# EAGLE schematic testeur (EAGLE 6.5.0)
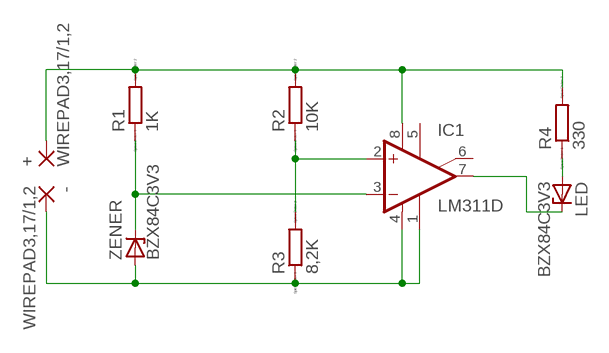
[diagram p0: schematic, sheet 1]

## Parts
+  WIREPAD3,17/1,2  [3,17/1,2]
-  WIREPAD3,17/1,2  [3,17/1,2]
IC1  LM311D  [SO08]
LED  BZX84C3V3  ZENER-DIODESOT23  [SOT23]
R1  1K  RR3216  [R3216]
R2  10K  RR3216  [R3216]
R3  8,2K  RR3216  [R3216]
R4  330  RR3216  [R3216]
ZENER  BZX84C3V3  ZENER-DIODESOT23  [SOT23]

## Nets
N$1: LED.1(A) R4.1
N$2: +.1(P) IC1.8(V+) R1.2 R2.2 R4.2
N$3: IC1.2(+IN) R2.1 R3.2
N$4: IC1.3(-IN) R1.1 ZENER.3(C)
N$5: -.1(P) IC1.1(GND) IC1.4(V-) R3.1 ZENER.1(A)
N$7: IC1.7(OUT) LED.3(C)
Unconnected: IC1.5(ON) IC1.6(ON/STR)

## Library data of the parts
+ - = wirepad:WIREPAD: Wire PAD connect wire on PCB
IC1 = linear:LM311: COMPARATOR
LED ZENER = diode:ZENER-DIODE: Z-Diode
R1-R4 = eagle-ltspice:R: RESISTOR, European symbol; SPICEMODEL: NONE; SPICEPREFIX: R

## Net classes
0 default: clearance 0.205 mm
